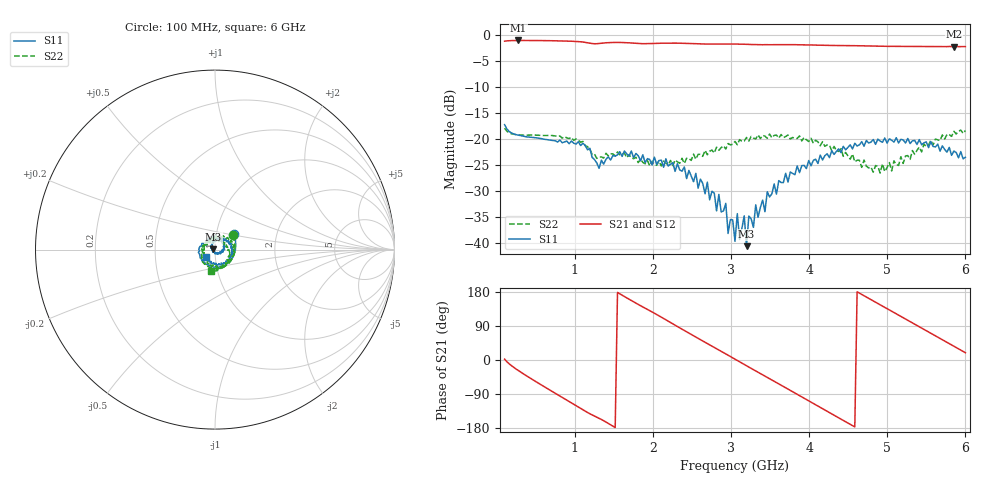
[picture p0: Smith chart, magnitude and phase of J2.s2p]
!Agilent Technologies,E8364B,MY43040379,A.07.50.67
!Agilent E8364B: A.07.50.67
!Date: Tuesday, March 24, 2026 10:35:52
!Correction: S11(Full 2 Port(1,2))
!S21(Full 2 Port(1,2))
!S12(Full 2 Port(1,2))
!S22(Full 2 Port(1,2))
!S2P File: Measurements: S11, S21, S12, S22:
# Hz S  dB  R 50
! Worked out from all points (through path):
!   201 points, 100 MHz to 6 GHz, reference 50 ohm
!   highest |S21| = -1.07 dB at 277 MHz (marker M1); lowest = -2.3 dB at 5.853 GHz (marker M2)
!   group delay of S21, straight-line fit = 325 ps
!   lowest |S11| = -40.7 dB at 3.197 GHz (marker M3), VSWR 1.02, Z = 49.1 + j0.157 ohm
!   |S11| at or under -10 dB: start of sweep to end of sweep
!   |S22| runs from -26.6 to -18.0 dB; largest |S21 - S12| = 0.004
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1e8  -17.30 38.6  -1.20 2.2  -1.22 2.3  -17.96 38.7
2.77e8  -19.30 -21.6  -1.07 -28.0  -1.10 -28.1  -19.24 -15.3
6.9e8  -20.28 -100.5  -1.11 -80.6  -1.14 -80.6  -19.36 -80.3
1.103e9  -20.87 178.4  -1.37 -131.5  -1.40 -131.5  -20.52 -144.4
1.3095e9  -25.70 151.8  -1.66 -153.6  -1.67 -153.6  -23.57 -156.7
1.575e9  -22.49 113.9  -1.46 174.6  -1.48 174.7  -23.10 169.6
2.0765e9  -24.19 49.6  -1.61 116.6  -1.62 116.6  -24.31 126.5
2.519e9  -28.27 -5.6  -1.67 63.9  -1.70 63.9  -22.96 98.1
2.932e9  -32.45 -89.6  -1.74 16.1  -1.76 16.1  -21.99 60.7
3.05e9  -39.76 -105.4  -1.76 2.2  -1.77 2.2  -20.52 46.3
3.0795e9  -34.42 -125.1  -1.76 -1.3  -1.78 -1.3  -21.16 44.0
3.109e9  -39.42 -168.4  -1.79 -4.8  -1.80 -4.8  -20.16 43.5
3.168e9  -34.85 -169.4  -1.80 -11.7  -1.82 -11.7  -20.44 36.2
3.1975e9  -40.69 170.0  -1.81 -15.2  -1.83 -15.2  -19.75 30.1
3.3155e9  -32.74 160.0  -1.86 -28.9  -1.88 -28.8  -20.04 17.3
3.699e9  -26.66 101.7  -1.88 -73.3  -1.89 -73.3  -19.57 -31.6
4.053e9  -24.16 78.3  -1.95 -115.0  -1.97 -114.9  -20.87 -87.0
4.5545e9  -21.97 33.1  -2.07 -173.2  -2.09 -173.1  -22.94 -173.0
5.0265e9  -20.02 -7.3  -2.21 132.1  -2.22 132.2  -24.59 68.1
5.4395e9  -21.17 -58.4  -2.21 84.4  -2.23 84.4  -22.52 -14.0
5.8525e9  -22.37 -107.4  -2.26 36.4  -2.26 36.4  -18.56 -78.2
6e9  -23.57 -139.5  -2.25 19.2  -2.26 19.3  -18.42 -99.7
